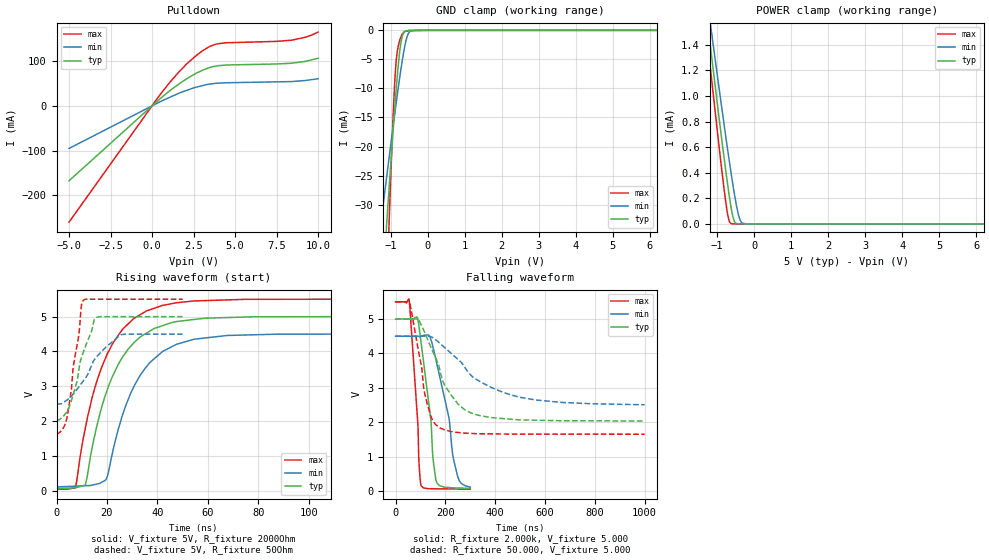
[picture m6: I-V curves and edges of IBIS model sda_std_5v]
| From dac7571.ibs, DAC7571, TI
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|   SDA_5V standard mode OPEN DRAIN MODEL
|   5v freq-400k,Rload=2Kohm, Cload = 15pF
[Model]   sda_std_5v
Model_type   I/O_open_drain
Polarity   Non-Inverting
Enable   Active-Low
Vinl = 1.5
Vinh = 3.5
Vmeas = 2.5
Vref = 5.0
Cref = 15pF
Rref = 2000
|   typ   min   max
|   (nom PVT)   (Fast PVT)   (Slow PVT)
|Average
C_comp   5.061e-12   5.040e-12   5.094e-12
|ON state : BUFFER OUTPUT TURNED LOW
|C_comp (ON state)   4.063e-10   3.336e-10   3.799e-10
|OFF state : BUFFER IN HIGH IMPEDANCE STATE
|C_comp   5.061e-12   5.094e-12   5.040e-12
|Where nom PVT is NOM Process, 5.0V,25C
|   Fast PVT is Strong Process, 5.5V, -40C
|   Slow PVT is Weak Process, 4.5V, 105C
[Model spec]
|   typ   min   max
Vinl   1.5   1.35   1.65
Vinh   3.5   3.15   3.85
[Voltage Range]   5   4.5   5.5
[Temperature Range]   25   105   -40
|Junction temperature
[Pullup Reference]   5   4.5   5.5
[Pulldown Reference]   0   0   0
[Power Clamp Reference]   5   4.5   5.5
[GND Clamp Reference]   0   0   0
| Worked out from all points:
|   slope of the pulldown table from 0 to 0.75 V, typ, clamps not added: 31.1 ohm
|   GND clamp passes 1 mA (typ) near -0.68 V on its own axis
|   POWER clamp passes 1 mA (typ) near -1.02 V on its own axis
|   falling waveform, R_fixture 2.000k, V_fixture 5.000: 20-80 % time 41.3ns typ, 63ns min, 26.3ns max; typ from 5 V to 0.079 V
|   rising waveform, V_fixture 5V, R_fixture 2000Ohm: 20-80 % time 14.3ns typ, 14.5ns min, 14.3ns max; typ from 0.073 V to 5 V
|   falling waveform, R_fixture 50.000, V_fixture 5.000: 20-80 % time 112ns typ, 211ns min, 55.8ns max; typ from 5 V to 2.03 V
|   rising waveform, V_fixture 5V, R_fixture 50Ohm: 20-80 % time 6.85ns typ, 11.3ns min, 4.33ns max; typ from 2.03 V to 5 V
[Pulldown]
|   Voltage   I(typ)   I(min)   I(max)
-5V       -167.6mA   -95.21mA   -260.1mA
632mV     20.56mA    11.88mA    32.24mA
1.567V    47.51mA    27.48mA    73.88mA
2.073V    60.23mA    34.53mA    93.27mA
3.03V     79.48mA    45.34mA    123mA
3.475V    85.81mA    48.85mA    133mA
3.866V    89.13mA    50.56mA    138.4mA
4.41V     91.14mA    51.64mA    141.1mA
7.49V     93.71mA    53.75mA    144.3mA
8.398V    95.44mA    54.36mA    146.9mA
9.239V    99.6mA     56.83mA    153.6mA
10V       106.6mA    60.8mA     165.1mA
[GND Clamp]
|   Voltage   I(typ)   I(min)   I(max)
-5V       -412.1mA   -229.4mA   -786.8mA
-1.266V   -48.89mA   -33.49mA   -75.73mA
-1.101V   -33mA      -25.04mA   -44.62mA
-1.04V    -27.31mA   -21.99mA   -33.44mA
-924.5mV  -16.82mA   -16.27mA   -14.04mA
-886mV    -13.47mA   -14.41mA   -8.932mA
-847.5mV  -10.29mA   -12.56mA   -5.324mA
-725mV    -2.321mA   -6.967mA   -1.233mA
-575mV    -62.02uA   -1.604mA   -142.6uA
-495.5mV  -53.37uA   -326.8uA   -12.8uA
-324.5mV  -34.76uA   -2.562uA   -8.377uA
10V       0A         0A         0A
[POWER Clamp]
|   Voltage   I(typ)   I(min)   I(max)
-5V       10.92mA    10.1mA     11.74mA
-1.335V   1.762mA    1.9mA      1.632mA
-1.265V   1.591mA    1.747mA    1.443mA
-1.238V   1.526mA    1.688mA    1.371mA
-1.15V    1.313mA    1.498mA    1.136mA
-748.5mV  378.2uA    647.3uA    135.5uA
-688mV    251.5uA    526.5uA    38.06uA
-622mV    128.1uA    396.8uA    2.687uA
-530mV    19.1uA     229.8uA    46.21nA
-401mV    1.196uA    49uA       34.99nA
-176mV    0A         0A         0A
10V       0A         0A         0A
[Ramp]
R_load = 2000
|   typ   min   max
dV/dt_r   2.95611/1.4249e-08   2.63191/1.44348e-08   3.26896/1.41366e-08
dV/dt_f   2.95255/4.11918e-08   2.59168/6.25614e-08   3.26871/2.62586e-08
[Falling Waveform]
R_fixture = 2.000k
V_fixture = 5.000
V_fixture_min = 4.500
V_fixture_max = 5.500
|  time   V(typ)   V(min)   V(max)
0s        5V         4.5V       5.5V
54.63ns   5V         4.5V       5.551V
87.01ns   5.05V      4.5V       2.206V
93.62ns   4.807V     4.5V       873.3mV
102.9ns   4.291V     4.498V     153mV
137.7ns   2.293V     4.49V      64.46mV
150.1ns   956.2mV    4.182V     63.52mV
165.6ns   240mV      3.699V     62.34mV
248.3ns   87.05mV    451.7mV    56.08mV
300ns     79.08mV    112.7mV    52.16mV
[Rising Waveform]
V_fixture = 5V
V_fixture_min = 4.5V
V_fixture_max = 5.5V
R_fixture = 2000Ohm
|   Time   V(typ)   V(min)   V(max)
0s        73.16mV    113.5mV    51.73mV
7.478ns   88.54mV    136.6mV    90.72mV
11.41ns   174.7mV    148.8mV    1.8V
15.55ns   1.729V     189.1mV    3.039V
19.56ns   2.78V      322.2mV    3.831V
27.57ns   3.978V     2.469V     4.73V
35.61ns   4.52V      3.557V     5.158V
42.4ns    4.747V     4.012V     5.322V
54.8ns    4.917V     4.351V     5.446V
150ns     5V         4.5V       5.5V
[Falling Waveform]
R_fixture = 50.000
V_fixture = 5.000
V_fixture_min = 4.500
V_fixture_max = 5.500
C_fixture = 0.000
|  time   V(typ)   V(min)   V(max)
0s        5V         4.5V       5.5V
55.81ns   5V         4.5V       5.482V
92.18ns   4.974V     4.5V       4.063V
123.4ns   4.495V     4.501V     2.64V
148.1ns   4.075V     4.464V     2.063V
180.6ns   3.421V     4.275V     1.825V
250.6ns   2.531V     3.824V     1.7V
342.4ns   2.184V     3.168V     1.663V
558.1ns   2.058V     2.65V      1.651V
1us       2.034V     2.506V     1.65V
[Rising Waveform]
V_fixture = 5V
V_fixture_min = 4.5V
V_fixture_max = 5.5V
R_fixture = 50Ohm
|   Time   V(typ)   V(min)   V(max)
0s        2.033V     2.492V     1.65V
4.178ns   2.282V     2.607V     2.114V
5.884ns   2.587V     2.717V     2.906V
6.654ns   2.772V     2.779V     3.569V
8.845ns   3.46V      2.982V     4.474V
9.878ns   3.817V     3.083V     5.318V
10.55ns   3.962V     3.149V     5.459V
15.64ns   4.967V     3.818V     5.496V
25.68ns   4.995V     4.479V     5.496V
50ns      4.995V     4.495V     5.496V
